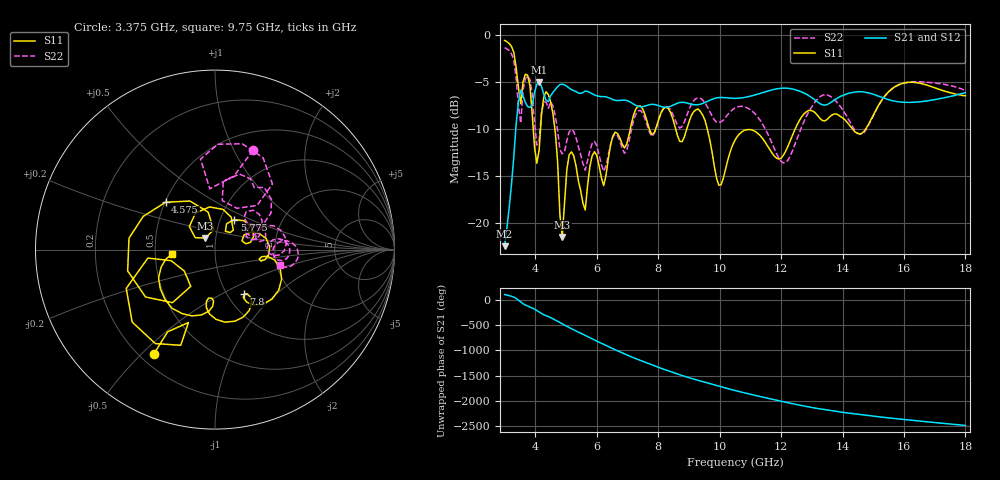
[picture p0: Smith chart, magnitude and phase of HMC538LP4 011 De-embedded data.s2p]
! Chelmsford, MA 01824
! http://www.hittite.com
! Tel: 978-250-3343
! Fax: 978-250-3373
! Device  :  HMC538LP4
! Description:  600 Analog Phase Shifter
! Frequency  :  6.0 GHz - 15.0 GHz
! Package  :  LP4  - 4x4 mm Quad Flatpack No-Lead (QFN) Plastic Package: 24 pin
! Ports  :  2 RF, 1 DC
!  Pin  3  = Rfin  = Port 1
!  Pin  16  = Rfout = Port 2
!  pin  21  = vCTL
! Voltages:  VCTL  = 0 to 5.0 Volts
! Currents :  Vb(V)  Vd(V)  Ib(mA)  Id(mA)
!  0.00  1.10  0.000000	0.488082
! Data:  The device was measured on evaluation board 111296-1.
!  Data was collected using a calibrated network analyzer.
!  The evaluation circuit board was modeled and simulated.This was use
!  to removed the evaluation board circuit from the measured data.
!  The reference plane is the center of the package pin.
! Misc:  Lot #
!Date Measured:  03 - 11 -2009
! Date:  03 - 17 -2009
! Note:
!  Hittite Microwave supplies this data as a sample of measured data at the
!  package pin for this package product.  Your particular data for this product
!  may vary.
!  Data was taken at 25 degrees C.
!  Hittite Microwave reserves the right to change this data at anytime.
# MHz S MA R 50
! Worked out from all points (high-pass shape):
!   201 points, 3 GHz to 18 GHz, reference 50 ohm
!   highest |S21| = -4.96 dB at 4.125 GHz (marker M1); lowest = -22.5 dB at 3 GHz (marker M2)
!   |S21| within 3 dB of the highest: 3.422 GHz to end of sweep
!   lowest |S11| = -21.5 dB at 4.875 GHz (marker M3), VSWR 1.18, Z = 44.6 + j5.83 ohm
!   |S11| at or under -10 dB: 4.637 GHz to 7.09 GHz (2.453 GHz wide, 41.8 % of centre); 8.571 GHz to 8.927 GHz (355.8 MHz wide, 4.07 % of centre); 9.6 GHz to 12.46 GHz (2.855 GHz wide, 25.9 % of centre)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
!   |S22| runs from -14.5 to -1.3 dB; largest |S21 - S12| = 0.0014
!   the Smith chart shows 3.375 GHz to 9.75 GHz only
!   S11 on the Smith chart (normalised r, x): 3.375 GHz: 0.26, -0.54; 4.575 GHz: 0.50, +0.31; 5.775 GHz: 1.17, +0.41; 7.8 GHz: 1.19, -0.65; 9.75 GHz: 0.61, -0.03
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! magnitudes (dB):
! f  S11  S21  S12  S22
! 3 GHz  -0.5  -22.5  -22.5  -1.3
! 3.375 GHz  -3.4  -9.5  -9.5  -4.5
! 3.825 GHz  -5.4  -7.7  -7.7  -4.8
! 4.125 GHz  -12.2  -5.0  -5.0  -11.2
! 4.275 GHz  -6.6  -6.3  -6.3  -7.1
! 4.575 GHz  -8.4  -6.1  -6.1  -7.5
! 4.875 GHz  -21.5  -5.2  -5.2  -12.6
! 5.1 GHz  -12.7  -5.6  -5.6  -10.3
! 5.55 GHz  -17.9  -6.1  -6.1  -13.7
! 5.775 GHz  -14.0  -6.1  -6.1  -12.3
! 6.225 GHz  -16.0  -6.5  -6.5  -14.5
! 7.35 GHz  -7.5  -7.6  -7.6  -8.0
! 7.8 GHz  -10.6  -7.4  -7.4  -10.8
! 8.025 GHz  -8.9  -7.5  -7.5  -8.9
! 9.75 GHz  -12.4  -6.8  -6.8  -8.6
! 10.05 GHz  -15.9  -6.6  -6.6  -9.2
! 10.5 GHz  -11.2  -6.7  -6.7  -7.7
! 12.07 GHz  -12.8  -5.6  -5.6  -13.6
! 13.05 GHz  -8.1  -6.8  -6.8  -7.4
! 14.62 GHz  -10.4  -6.0  -6.0  -10.5
! 15.53 GHz  -5.9  -6.9  -6.9  -6.0
! 18 GHz  -6.4  -6.1  -6.1  -5.9
